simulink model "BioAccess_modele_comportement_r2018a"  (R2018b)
settings: Solver=ode23  StartTime=0.0  StopTime=0.2  RelTol=1e-3  EnableMultiTasking=on
undefined symbols (not defined in the file): sigbuilder_block

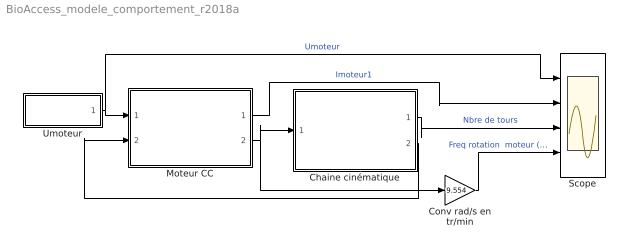
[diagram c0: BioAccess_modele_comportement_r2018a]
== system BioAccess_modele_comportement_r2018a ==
  Chaine cinématique : Subsystem
  Conv rad/s en tr/min : Gain  Gain=9.554
  Moteur CC : Subsystem
  Scope : Scope  NumInputPorts=4
  Umoteur : Subsystem  Tag=STV Subsys  LoadFcn=sigbuilder_block('load',[437.25 117.75 550.5 399.75 ]);  StartFcn=sigbuilder_block('start');  StopFcn=sigbuilder_block('stop');  ClipboardFcn=sigbuilder_block('clipboard');  mask(Sigbuilder block){tuvar=[0:10]}
      mask help: Sigbuilder GUI
      mask init:
      | if ~strcmp(get_param(bdroot(gcbh),'SimulationStatus'),'stopped') tuvar = sigbuilder_block('maskInit'); end
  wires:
  Conv rad/s en tr/min/1 -> Scope/4  "Freq rotation  moteur (tr/min)"
  Umoteur/1(Signal 1) -> Scope/1, Moteur CC/1(Umoteur)  "Umoteur"
  Chaine cinématique/1(Tours) -> Scope/3  "Nbre de tours"
  Chaine cinématique/2(Cr) -> Moteur CC/2(Cr)
  Moteur CC/2(Omega moteur) -> Chaine cinématique/1(Omega), Conv rad/s en tr/min/1
  Moteur CC/1(Imoteur) -> Scope/2  "Imoteur1"

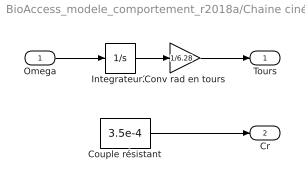
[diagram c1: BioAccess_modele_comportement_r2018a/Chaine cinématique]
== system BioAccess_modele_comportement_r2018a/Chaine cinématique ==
  Omega : Inport
  Conv rad en tours : Gain  Gain=1/6.28
  Couple résistant : Constant  Value=3.5e-4
  Integrateur2 : Integrator
  Tours : Outport
  Cr : Outport  Port=2
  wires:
  Omega/1 -> Integrateur2/1
  Integrateur2/1 -> Conv rad en tours/1
  Conv rad en tours/1 -> Tours/1
  Couple résistant/1 -> Cr/1

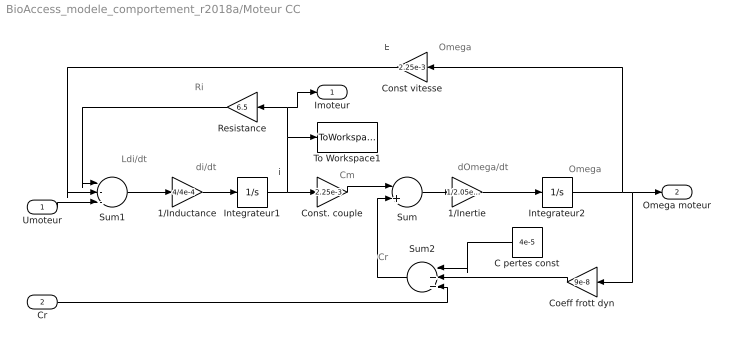
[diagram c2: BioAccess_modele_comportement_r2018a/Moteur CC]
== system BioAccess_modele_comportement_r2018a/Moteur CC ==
  note: di/dt
  note: i
  note: dOmega/dt
  note: Omega
  note: Omega
  note: E
  note: Cr
  note: Cm
  note: Ri
  note: Ldi/dt
  Umoteur : Inport
  Cr : Inport  Port=2
  1/Inductance : Gain  Gain=4/4e-4
  1/Inertie : Gain  Gain=1/2.05e-8
  C pertes const : Constant  Value=4e-5  VectorParams1D=off
  Coeff frott dyn : Gain  Gain=9e-8
  Const vitesse : Gain  Gain=2.25e-3
  Const. couple : Gain  Gain=2.25e-3
  Integrateur1 : Integrator  LimitOutput=on  LowerSaturationLimit=0
  Integrateur2 : Integrator  LimitOutput=on  LowerSaturationLimit=0
  Resistance : Gain  Gain=6.5
  Sum : Sum  Inputs=|+-
  Sum1 : Sum  Inputs=|--+
  Sum2 : Sum  Inputs=|+++
  To Workspace1 : ToWorkspace  VariableName=Imot1  SampleTime=8e-5
  Imoteur : Outport
  Omega moteur : Outport  Port=2
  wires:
  1/Inductance/1 -> Integrateur1/1
  Integrateur1/1 -> Const. couple/1, Resistance/1, Imoteur/1, To Workspace1/1
  1/Inertie/1 -> Integrateur2/1
  Integrateur2/1 -> Const vitesse/1, Coeff frott dyn/1, Omega moteur/1
  Sum/1 -> 1/Inertie/1
  Sum1/1 -> 1/Inductance/1
  Resistance/1 -> Sum1/1
  C pertes const/1 -> Sum2/1
  Coeff frott dyn/1 -> Sum2/2
  Const vitesse/1 -> Sum1/2
  Umoteur/1 -> Sum1/3
  Sum2/1 -> Sum/2
  Const. couple/1 -> Sum/1
  Cr/1 -> Sum2/3

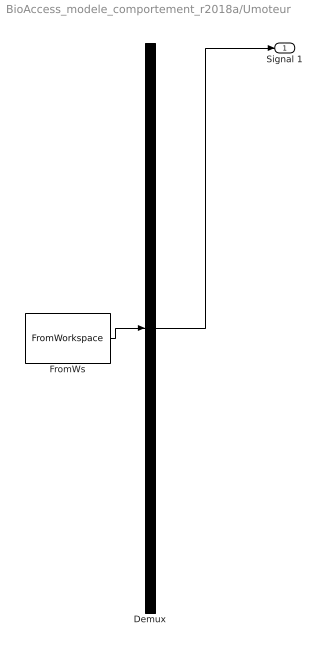
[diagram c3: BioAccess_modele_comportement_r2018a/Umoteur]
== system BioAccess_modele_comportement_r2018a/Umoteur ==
  Demux : Demux  Tag=STV Demux  Outputs=1
  FromWs : FromWorkspace  Tag=STV FromWs  VariableName=tuvar  SampleTime=0
  Signal 1 : Outport  Tag=STV Outport
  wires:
  Demux/1 -> Signal 1/1
  FromWs/1 -> Demux/1
